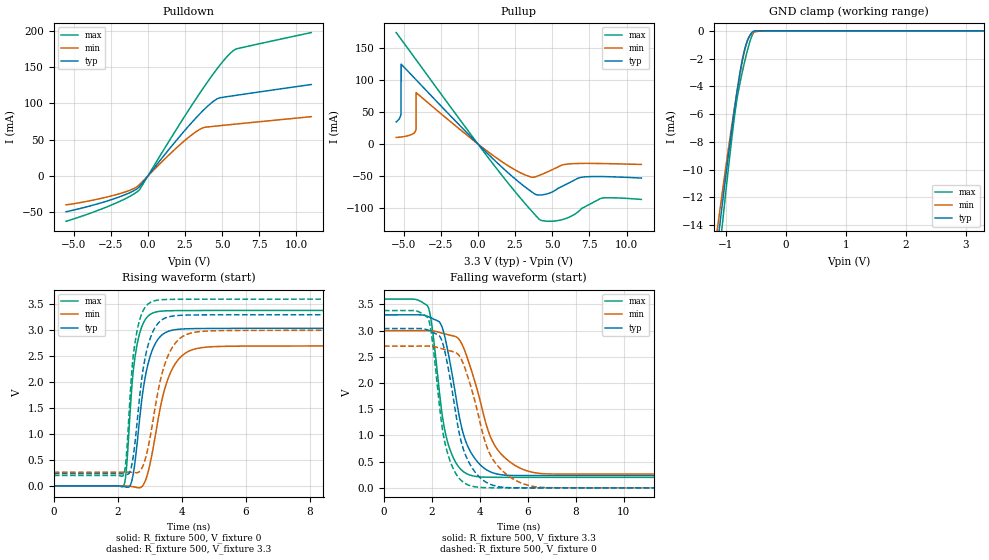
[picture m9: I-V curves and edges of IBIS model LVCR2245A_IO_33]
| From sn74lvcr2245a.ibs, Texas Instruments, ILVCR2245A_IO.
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[Model]   LVCR2245A_IO_33
Model_type  I/O
Vinl=0.8
Vinh=2.0
Enable   Active-Low
Vref =   0
Rref =   500
Cref =   50p
Vmeas =   1.5
| variable   typ   min   max
C_comp   5.77pF   5.39pF   7.14pF
| C_pullup   4.64pF   4.30pF   6.71pF
| C_pulldown   4.30pF   3.81pF   5.46pF
| C_tri-state   5.77pF   5.39pF   7.14pF
[Temperature Range]   40   100   -40
| Ambient temperature   25   85   -40
[Voltage range]   3.3   3   3.6
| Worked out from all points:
|   slope of the pulldown table from 0 to 0.495 V, typ, clamps not added: 38.3 ohm
|   slope of the pullup table from 0 to 0.495 V, typ, clamps not added: 43.1 ohm
|   GND clamp passes 1 mA (typ) near -0.67 V on its own axis
|   rising waveform, R_fixture 500, V_fixture 0: 20-80 % time 412ps typ, 584ps min, 286ps max; typ from 0 V to 3.04 V
|   falling waveform, R_fixture 500, V_fixture 3.3: 20-80 % time 816ps typ, 1.12ns min, 602ps max; typ from 3.3 V to 0.234 V
|   rising waveform, R_fixture 500, V_fixture 3.3: 20-80 % time 396ps typ, 563ps min, 279ps max; typ from 0.234 V to 3.3 V
|   falling waveform, R_fixture 500, V_fixture 0: 20-80 % time 800ps typ, 1.08ns min, 599ps max; typ from 3.04 V to 0 V
[GND Clamp]
| LVCR2245A_IO_33
|   Voltage   I(typ)   I(min)   I(max)
-5.5V     -191mA     -172.6mA   -219.2mA
-1.155V   -15.81mA   -14.6mA    -17.82mA
-1.115V   -14.36mA   -13.31mA   -16.15mA
-1.075V   -12.94mA   -12.03mA   -14.49mA
-1.04V    -11.7mA    -10.93mA   -13.06mA
-925mV    -7.771mA   -7.427mA   -8.522mA
-850mV    -5.367mA   -5.277mA   -5.881mA
-805mV    -4.027mA   -4.064mA   -4.603mA
-740mV    -2.332mA   -2.466mA   -3.187mA
-635mV    -627.2uA   -606.9uA   -1.272mA
-525mV    -20.03uA   -86.68uA   -33.12uA
3.3V      65.9pA     44.07nA    -1.765nA
[Pulldown]
| LVCR2245A_IO_33
|   Voltage   I(typ)   I(min)   I(max)
-5.5V     -49.08mA   -39.61mA   -62.2mA
-2.2V     -30.71mA   -25.97mA   -37.66mA
-1.115V   -21.93mA   -18.74mA   -26.78mA
-590mV    -15.23mA   -12.3mA    -19.43mA
1.815V    46.38mA    36.59mA    60.63mA
3.335V    81.96mA    62.14mA    108.9mA
3.82V     92.07mA    67mA       123.5mA
4.64V     105.8mA    68.83mA    146.9mA
5.275V    109mA      70.15mA    162.9mA
5.75V     110.4mA    71.12mA    172.3mA
6.01V     111.2mA    71.66mA    175.2mA
11V       125.9mA    81.65mA    197.3mA
[Pullup]
| LVCR2245A_IO_33
|   Voltage   I(typ)   I(min)   I(max)
-5.5V     34.62mA    10.2mA     174.7mA
-5.18V    47.43mA    10.96mA    164.5mA
-5.175V   49.33mA    10.98mA    164.4mA
-5.17V    125.2mA    10.99mA    164.2mA
-4.185V   101.2mA    21.01mA    132.8mA
-4.165V   100.7mA    23.5mA     132.2mA
-4.16V    100.6mA    80.49mA    132mA
1.67V     -37.57mA   -28.61mA   -50.75mA
4.155V    -79.99mA   -48.93mA   -118.6mA
6.96V     -52.23mA   -30.49mA   -101.7mA
8.385V    -51.06mA   -30.68mA   -84.72mA
11V       -53.45mA   -32.08mA   -86.89mA
[Ramp]
| LVCR2245A_IO_33
| variable   typ   min   max
dV/dt_r   1.84/4.18E-10   1.64/5.92E-10   2.04/2.90E-10
dV/dt_f   1.84/8.17E-10   1.64/1.13E-09   2.04/6.03E-10
R_load = 500
[Rising Waveform]
| LVCR2245A_IO_33
R_fixture =   500
C_fixture =   0
L_fixture =   0
V_fixture =   0
V_fixture_min = 0
V_fixture_max = 0
|   Time   V(typ)   V(min)   V(max)
0s        937.6pV    2.878nV    27.68nV
2.18ns    -10.58mV   -859.3uV   -2.201mV
2.275ns   -26.71mV   -2.38mV    391.8mV
2.425ns   73.24mV    -11.66mV   1.819V
2.62ns    932.7mV    -35.69mV   2.785V
2.91ns    2.27V      194.2mV    3.251V
3.33ns    2.882V     1.524V     3.367V
3.915ns   3.02V      2.455V     3.379V
5.03ns    3.035V     2.685V     3.381V
50ns      3.038V     2.699V     3.382V
[Falling Waveform]
| LVCR2245A_IO_33
R_fixture =   500
C_fixture =   0
L_fixture =   0
V_fixture =   3.3
V_fixture_min = 3
V_fixture_max = 3.6
|   Time   V(typ)   V(min)   V(max)
0s        3.3V       3V         3.6V
1.83ns    3.27V      3.001V     3.463V
2.01ns    3.232V     2.997V     3.056V
2.34ns    3.146V     2.962V     1.716V
2.88ns    2.068V     2.899V     585.5mV
3.305ns   1.034V     2.686V     311.6mV
3.835ns   532.8mV    1.955V     218mV
4.75ns    261mV      719.1mV    200.8mV
6.59ns    234.2mV    271.1mV    200.3mV
50ns      234.1mV    261.4mV    200.1mV
[Rising Waveform]
| LVCR2245A_IO_33
R_fixture =   500
C_fixture =   0
L_fixture =   0
V_fixture =   3.3
V_fixture_min = 3
V_fixture_max = 3.6
|   Time   V(typ)   V(min)   V(max)
0s        234mV      261.3mV    200.1mV
2.175ns   230.1mV    264.2mV    204mV
2.265ns   220.5mV    265.2mV    583.4mV
2.415ns   351.4mV    261.4mV    2.046V
2.605ns   1.256V     255.1mV    3.007V
2.885ns   2.569V     586.6mV    3.47V
3.305ns   3.165V     1.976V     3.585V
3.87ns    3.284V     2.805V     3.597V
4.91ns    3.297V     2.988V     3.599V
50ns      3.3V       3V         3.6V
[Falling Waveform]
| LVCR2245A_IO_33
R_fixture =   500
C_fixture =   0
L_fixture =   0
V_fixture =   0
V_fixture_min = 0
V_fixture_max = 0
|   Time   V(typ)   V(min)   V(max)
0s        3.04V      2.703V     3.383V
1.83ns    3.009V     2.704V     3.243V
2.01ns    2.971V     2.7V       2.828V
2.335ns   2.883V     2.665V     1.479V
2.885ns   1.734V     2.597V     369.1mV
3.28ns    782.1mV    2.398V     117.6mV
3.83ns    281.8mV    1.586V     17.84mV
4.67ns    32.84mV    458.6mV    828.2uV
6.56ns    197.6uV    8.973mV    185.9uV
50ns      24.96uV    46.23uV    7.621uV
